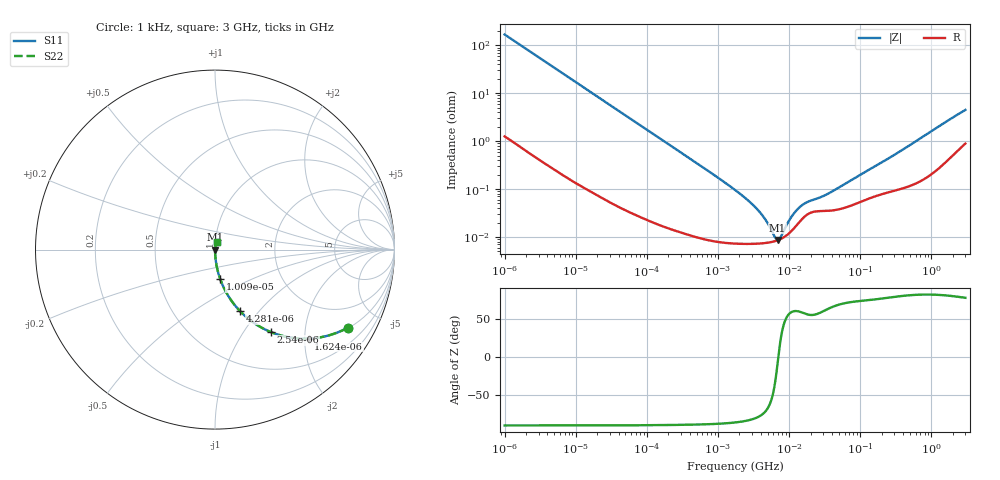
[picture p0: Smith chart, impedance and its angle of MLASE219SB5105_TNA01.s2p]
! MLASE219SB5105_TNA01  S-PARAMETER MODEL  ( Standard Model )
! Model Generated by TAIYO YUDEN Corporation (http://www.ty-top.com)
! Version 1.0
! TAIYO YUDEN Control No. 220601
! Copyright(c) 2009 TAIYO YUDEN CO.,LTD. All Rights Reserved.
! Product Description (link to TY-COMPAS)
! https://ds.yuden.co.jp/TYCOMPAS/or/detail?pn=MLASE219SB5105KTNA01&u=M
! Products Name : Multilayer Ceramic Capacitors
! Characteristics :
!  Capacitance : 1 [uF] , Rated Voltage : 16 [V] , TCC : B / X5R
!  Case Size : 2.0 x 1.25 / 0.079 x 0.049 [mm/inch] , Thickness : 0.85 / 0.033 [mm/inch]
!  (Conditions: Temperature = 25 [degC] , DC Bias Voltage = 0 [V])
! External Node Assignments :
!  1  o---| |---o  2
! GND o---------o GND
! Frequency Range : 1kHz  -  3GHz  [ 401 STEP ]
# MHZ S RI R 50
! Freq[MHz].  S11 Real  S11 Imag  S21 Real  S21 Imag  S12 Real  S12 Imag  S22 Real  S22 Imag
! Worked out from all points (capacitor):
!   401 points, 1 kHz to 3 GHz, reference 50 ohm
!   read as one part in series: C = 939 nF near 1.077 kHz
!   lowest |Z| = 8.58 mohm at 6.882 MHz (marker M1)
!   series resonance near 7.03 MHz, so ESL is about 550 pH
!   S11 on the Smith chart (normalised r, x): 1 kHz: 1.03, -3.38; 1.624 kHz: 1.02, -2.09; 2.54 kHz: 1.01, -1.34; 4.281 kHz: 1.01, -0.80; 10.09 kHz: 1.00, -0.34; 3 GHz: 1.02, +0.09
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0.001  0.7397 -0.4351  0.2603 0.4351  0.2603 0.4351  0.7397 -0.4351
0.001624  0.5219 -0.4958  0.4781 0.4958  0.4781 0.4958  0.5219 -0.4958
0.00254  0.3108 -0.4592  0.6892 0.4592  0.6892 0.4592  0.3108 -0.4592
0.004281  0.1387 -0.3419  0.8613 0.3419  0.8613 0.3419  0.1387 -0.3419
0.010091  0.0291 -0.1644  0.9709 0.1644  0.9709 0.1644  0.0291 -0.1644
0.01216  0.0205 -0.1378  0.9795 0.1378  0.9795 0.1378  0.0205 -0.1378
0.033275  0.00315 -0.0515  0.9968 0.0515  0.9968 0.0515  0.00315 -0.0515
0.147855  0.000316 -0.0117  0.9997 0.0117  0.9997 0.0117  0.000316 -0.0117
1.732051  7.34e-05 -0.000956  0.9999 0.000956  0.9999 0.000956  7.34e-05 -0.000956
3.651041  7.25e-05 -0.000356  0.9999 0.000356  0.9999 0.000356  7.25e-05 -0.000356
4.739869  7.49e-05 -0.000206  0.9999 0.000206  0.9999 0.000206  7.49e-05 -0.000206
6.153411  8.07e-05 -6.86e-05  0.9999 6.86e-05  0.9999 6.86e-05  8.07e-05 -6.86e-05
6.881678  8.51e-05 -1.1e-05  0.9999 1.1e-05  0.9999 1.1e-05  8.51e-05 -1.1e-05
7.414467  8.91e-05 2.76e-05  0.9999 -2.76e-05  0.9999 -2.76e-05  8.91e-05 2.76e-05
7.988506  9.41e-05 6.65e-05  0.9999 -6.65e-05  0.9999 -6.65e-05  9.41e-05 6.65e-05
10.37087  0.000126 0.000207  0.9999 -0.000207  0.9999 -0.000207  0.000126 0.000207
12.97096  0.000181 0.000325  0.9998 -0.000325  0.9998 -0.000325  0.000181 0.000325
16.22291  0.00026 0.000418  0.9997 -0.000418  0.9997 -0.000418  0.00026 0.000418
21.06097  0.000329 0.000485  0.9997 -0.000485  0.9997 -0.000485  0.000329 0.000485
36.84432  0.000353 0.00075  0.9996 -0.00075  0.9996 -0.00075  0.000353 0.00075
256.0921  0.000882 0.00438  0.9991 -0.00438  0.9991 -0.00438  0.000882 0.00438
3000  0.0107 0.0432  0.9893 -0.0432  0.9893 -0.0432  0.0107 0.0432
